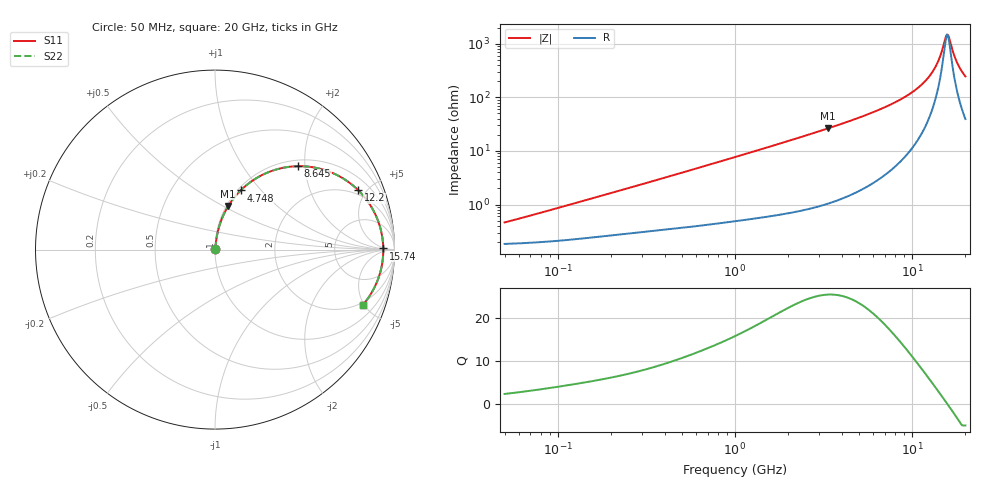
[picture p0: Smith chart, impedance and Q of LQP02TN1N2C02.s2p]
!Murata Part Number: LQP02TN1N2C02
!These Parameters are Measured in Series Mode Connection
!  o--[Z]--o
!Port1  Port2
!  o-------o
!Freq. Start=50[MHz] Stop=20[GHz], 401[Steps]
# Hz S RI R 50
!Freq.(Hz) S11(Real) S11(Imag) S21(Real) S21(Imag) S12(Real) S12(Imag) S22(Real) S22(Imag)
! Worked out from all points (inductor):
!   401 points, 50 MHz to 20 GHz, reference 50 ohm
!   read as one part in series: L = 1.34 nH near 68.48 MHz
!   highest Q = 25.4 at 3.364 GHz (marker M1), where L = 1.25 nH
!   self-resonance near 15.81 GHz
!   S11 on the Smith chart (normalised r, x): 50 MHz: 1.00, +0.01; 4.748 GHz: 1.03, +0.78; 8.645 GHz: 1.13, +1.84; 12.2 GHz: 1.69, +4.41; 15.74 GHz: 31, +3; 20 GHz: 1.79, -4.86
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5e7  0.00185 0.00424  0.9981 -0.00424  0.9981 -0.00424  0.00185 0.00424
1.364002e8  0.00244 0.0112  0.9976 -0.0112  0.9976 -0.0112  0.00244 0.0112
3.721004e8  0.00413 0.0291  0.9959 -0.0291  0.9959 -0.0291  0.00413 0.0291
1e9  0.0106 0.0755  0.9894 -0.0755  0.9894 -0.0755  0.0106 0.0755
2.728004e9  0.0502 0.199  0.9498 -0.199  0.9498 -0.199  0.0502 0.199
3.364474e9  0.0738 0.2425  0.9262 -0.2425  0.9262 -0.2425  0.0738 0.2425
4.748272e9  0.1429 0.3297  0.8571 -0.3297  0.8571 -0.3297  0.1429 0.3297
6.034176e9  0.2294 0.3973  0.7706 -0.3973  0.7706 -0.3973  0.2294 0.3973
7.442007e9  0.347 0.448  0.653 -0.448  0.653 -0.448  0.347 0.448
8.644534e9  0.4622 0.4647  0.5378 -0.4647  0.5378 -0.4647  0.4622 0.4647
1.050288e10  0.6487 0.4296  0.3513 -0.4296  0.3513 -0.4296  0.6487 0.4296
1.220001e10  0.7985 0.3304  0.2015 -0.3304  0.2015 -0.3304  0.7985 0.3304
1.295331e10  0.8505 0.2695  0.1495 -0.2695  0.1495 -0.2695  0.8505 0.2695
1.375312e10  0.8929 0.1973  0.1071 -0.1973  0.1071 -0.1973  0.8929 0.1973
1.438523e10  0.9164 0.137  0.0836 -0.137  0.0836 -0.137  0.9164 0.137
1.527346e10  0.9346 0.051  0.0654 -0.051  0.0654 -0.051  0.9346 0.051
1.573793e10  0.9375 0.0067  0.0625 -0.0067  0.0625 -0.0067  0.9375 0.0067
1.621653e10  0.9363 -0.0377  0.0637 0.0377  0.0637 0.0377  0.9363 -0.0377
1.721783e10  0.9213 -0.1247  0.0787 0.1247  0.0787 0.1247  0.9213 -0.1247
1.800918e10  0.8998 -0.1863  0.1002 0.1863  0.1002 0.1863  0.8998 -0.1863
1.912117e10  0.8596 -0.2607  0.1404 0.2607  0.1404 0.2607  0.8596 -0.2607
2e10  0.8225 -0.3095  0.1775 0.3095  0.1775 0.3095  0.8225 -0.3095
